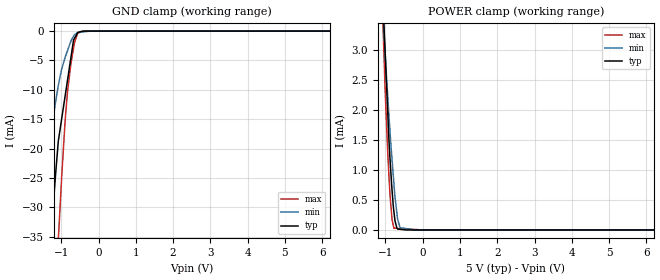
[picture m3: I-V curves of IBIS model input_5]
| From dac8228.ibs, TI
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|   input_5 Model
[Model]   input_5
Model_type   Input
Vinl = 0.8
Vinh = 3.8
|   typ   min   max
|   (nom PVT)   (Fast PVT)   (slow PVT)
|C_comp from frequency method(F=50MHz)
|Average
|C_comp   4.586e-12   3.935e-12   5.094e-12
|C_comp from L-C Tank method(L=1nH)
|Resonant Frequency(Hz)   2.82e9   2.84e9   2.8e9
C_comp   3.188e-12  3.144e-12   3.234e-12
| Where nom  PVT is Nominal Process,  5V,  33C
|   Fast PVT is Strong Process,   5.5V,  -40C
|   Slow PVT is Weak Process,   4.5V,  113C
[Voltage Range]   5   4.5   5.5
|Ambient Temperature   25   105   -40
|Junction Temperature
[Temperature Range]   33   113   -40
[Power Clamp Reference]   5   4.5   5.5
[GND Clamp Reference]   0   0   0
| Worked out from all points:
|   GND clamp passes 1 mA (typ) near -0.62 V on its own axis
|   POWER clamp passes 1 mA (typ) near -0.86 V on its own axis
[GND Clamp]
|   Voltage   I(typ)   I(min)   I(max)
-5V       -466.2mA   -327.1mA   -581.8mA
-1.56V    -62.89mA   -33.62mA   -100mA
-1.373V   -44.06mA   -22.58mA   -73.94mA
-1.269V   -34.46mA   -17.29mA   -60.01mA
-1.08V    -18.75mA   -9.263mA   -35.55mA
-994.5mV  -15.16mA   -6.584mA   -25.52mA
-907.5mV  -11.5mA    -4.706mA   -16.36mA
-830.5mV  -8.266mA   -3.284mA   -10.16mA
-742.5mV  -4.568mA   -1.734mA   -5.617mA
-670mV    -1.521mA   -846.2uA   -2.906mA
-553.5mV  -239.4uA   -198.9uA   -334.8uA
10V       0A         0A         0A
[POWER Clamp]
|   Voltage   I(typ)   I(min)   I(max)
-5V       81.16mA    67.53mA    99.14mA
-1.073V   3.867mA    3.699mA    3.539mA
-1.053V   3.588mA    3.45mA     3.17mA
-1.012V   3.001mA    2.994mA    2.396mA
-946mV    2.057mA    2.289mA    1.382mA
-907.5mV  1.506mA    1.911mA    903uA
-825mV    674.1uA    1.184mA    180.7uA
-775.5mV  315.9uA    789.6uA    30.48uA
-679.5mV  22.42uA    203.8uA    26.71uA
-607.5mV  10.87uA    37.96uA    23.88uA
-202.5mV  2.274nA    0A         7.959uA
10V       0A         0A         0A
